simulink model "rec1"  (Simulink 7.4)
settings: Solver=ode15s  StartTime=0.0  StopTime=0.05  MaxStep=1e-4  RelTol=1e-5  AbsTol=1e-5

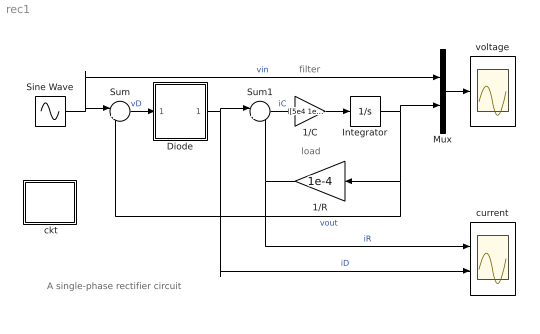
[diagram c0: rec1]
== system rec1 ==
  note: A single-phase rectifier circuit
  note: filter
  note: load
  " ckt" : Subsystem
  1/C : Gain  Gain=[5e4 1e5 3e5 1e10]  ParameterDataType=sfix(16)  ParameterScaling=2^0  OutDataType=sfix(16)  OutScaling=2^0
  1/R : Gain  Gain=1e-4  ParameterDataType=sfix(16)  ParameterScaling=2^0  OutDataType=sfix(16)  OutScaling=2^0
  Diode : Subsystem
  Integrator : Integrator
  Mux : Mux  Inputs=2
  Sine Wave : Sin  Amplitude=24  Bias=0  Frequency=2*pi*60  Phase=0  Samples=10  SampleTime=0
  Sum : Sum  Inputs=|+-  OutDataType=sfix(16)  OutScaling=2^0
  Sum1 : Sum  Inputs=|+-  OutDataType=sfix(16)  OutScaling=2^0
  current : Scope  NumInputPorts=2
  voltage : Scope
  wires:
  1/C/1 -> Integrator/1
  Integrator/1 -> Mux/2, 1/R/1, Sum/2  "vout"
  Mux/1 -> voltage/1
  Sine Wave/1 -> Sum/1, Mux/1  "vin"
  Sum/1 -> Diode/1(vD)  "vD"
  1/R/1 -> Sum1/2, current/1  "iR"
  Diode/1(iD) -> Sum1/1, current/2  "iD"
  Sum1/1 -> 1/C/1  "iC"

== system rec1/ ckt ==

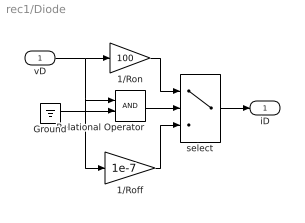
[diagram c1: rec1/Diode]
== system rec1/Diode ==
  vD : Inport  OutDataType=sfix(16)  OutScaling=2^0
  1/Roff : Gain  Gain=1e-7  ParameterDataType=sfix(16)  ParameterScaling=2^0  OutDataType=sfix(16)  OutScaling=2^0
  1/Ron : Gain  Gain=100  ParameterDataType=sfix(16)  ParameterScaling=2^0  OutDataType=sfix(16)  OutScaling=2^0
  Ground : Ground
  Relational Operator : RelationalOperator
  select : Switch  Threshold=0.5
  iD : Outport
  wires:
  Ground/1 -> Relational Operator/2
  Relational Operator/1 -> select/2
  1/Ron/1 -> select/1
  1/Roff/1 -> select/3
  select/1 -> iD/1
  vD/1 -> 1/Ron/1, Relational Operator/1, 1/Roff/1
